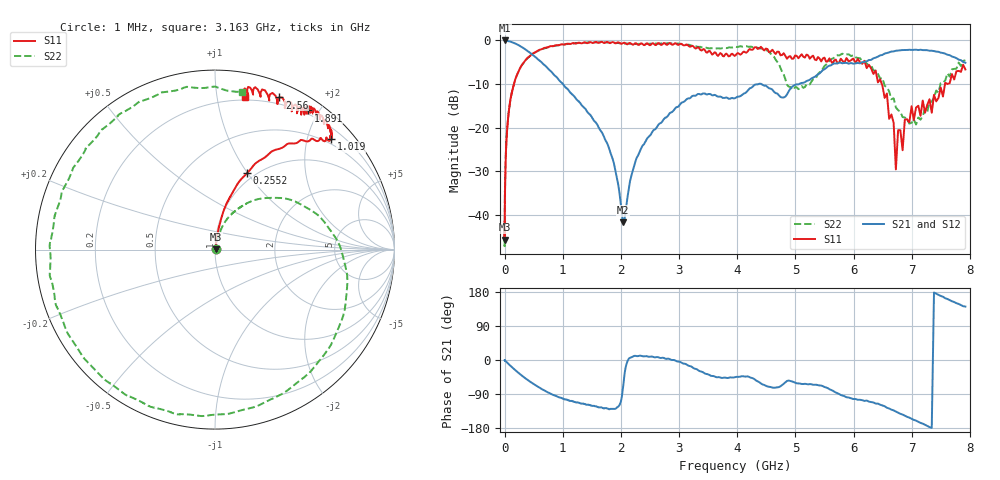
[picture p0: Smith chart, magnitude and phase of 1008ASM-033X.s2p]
!s-Parameter Generated by FASTRON Sdn. Bhd.
!FASTRON P/N : 1008ASM-033X
!Keysight Technologies: E5071C_MY46733604_B.14.02
!Date: Tue Nov 21 11:22:15 2023
!Version  :Rev00  Wed Nov 22 15:47:42 2023
!Data & Calibration Information:
!Freq  S11:SOLT2(ON)  S21:SOLT2(ON)  S12:SOLT2(ON)  S22:SOLT2(ON)
!PortZ  Port1:50+j0  Port2:50+j0
!When reading reference impedance value at option line is always used.
! Remarks : This data is being provided solely for informational purposes.
# Hz S dB R 50
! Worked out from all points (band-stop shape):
!   1599 points, 1 MHz to 7.923 GHz, reference 50 ohm
!   highest |S21| = -0.03 dB at 6.301 MHz (marker M1); lowest = -41.7 dB at 2.04 GHz (marker M2)
!   |S21| within 3 dB of the highest: start of sweep to 454.7 MHz; 6.535 GHz to 7.568 GHz (1.033 GHz wide, 14.6 % of centre)
!   lowest |S11| = -45.7 dB at 1.586 MHz (marker M3), VSWR 1.01, Z = 50.5 + j0.193 ohm
!   |S11| at or under -10 dB: start of sweep to 161.5 MHz; 6.486 GHz to 7.573 GHz (1.087 GHz wide, 15.5 % of centre)
!   |S22| runs from -47.2 to -0.4 dB; largest |S21 - S12| = 0.014
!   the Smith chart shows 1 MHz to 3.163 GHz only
!   S11 on the Smith chart (normalised r, x): 1 MHz: 1.01, +0.00; 255.2 MHz: 0.92, +1.00; 1.019 GHz: 0.40, +2.44; 1.891 GHz: 0.16, +1.86; 2.56 GHz: 0.14, +1.50; 3.163 GHz: 0.18, +1.20
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1000000  -43.30 9.7  -0.05 -0.3  -0.05 -0.1  -43.50 15.6
1586469  -45.70 21.6  -0.05 -0.3  -0.05 -0.2  -44.40 9.4
4479405  -38.70 60.4  -0.06 -0.8  -0.06 -0.7  -38.90 64.4
6301378  -36.00 58.2  -0.03 -1.1  -0.08 -1.0  -38.40 65.5
1.99485e7  -27.10 78.9  -0.07 -3.2  -0.08 -3.1  -26.90 76.2
8.901281e7  -14.60 78.4  -0.25 -13.5  -0.26 -13.4  -14.70 68.3
2.552003e8  -6.71 67.2  -1.22 -36.0  -1.23 -36.0  -6.69 38.5
3.985133e8  -3.99 60.0  -2.47 -52.6  -2.47 -52.7  -4.03 14.1
6.665231e8  -1.85 49.0  -5.46 -78.8  -5.46 -78.9  -1.91 -26.9
1.019114e9  -0.98 43.7  -10.30 -103.0  -10.30 -103.0  -0.95 -72.4
1.784248e9  -0.47 56.1  -24.30 -129.0  -24.30 -129.0  -0.52 -147.0
1.890772e9  -0.61 56.3  -28.90 -129.0  -28.90 -130.0  -0.58 -159.0
2.039907e9  -0.60 56.8  -41.70 -69.1  -41.70 -69.4  -0.67 -173.0
2.560258e9  -0.72 67.1  -20.60 7.9  -20.70 7.8  -0.81 136.0
3.162936e9  -1.26 78.9  -13.30 -15.2  -13.30 -15.2  -1.00 80.2
3.872345e9  -3.61 68.8  -13.40 -46.1  -13.40 -46.3  -1.61 4.3
4.548578e9  -2.70 113.0  -11.00 -70.8  -11.00 -71.0  -2.68 -49.1
5.052431e9  -4.11 146.0  -10.10 -61.8  -10.10 -62.0  -11.20 -99.1
5.808211e9  -4.67 148.0  -5.27 -93.8  -5.25 -94.0  -3.06 -143.0
6.534915e9  -13.20 146.0  -3.03 -122.0  -3.01 -123.0  -10.40 -162.0
7.074683e9  -15.40 -107.0  -2.15 -160.0  -2.14 -161.0  -19.30 -173.0
7.92289e9  -6.68 -61.4  -5.14 141.0  -5.13 140.0  -4.58 126.0
